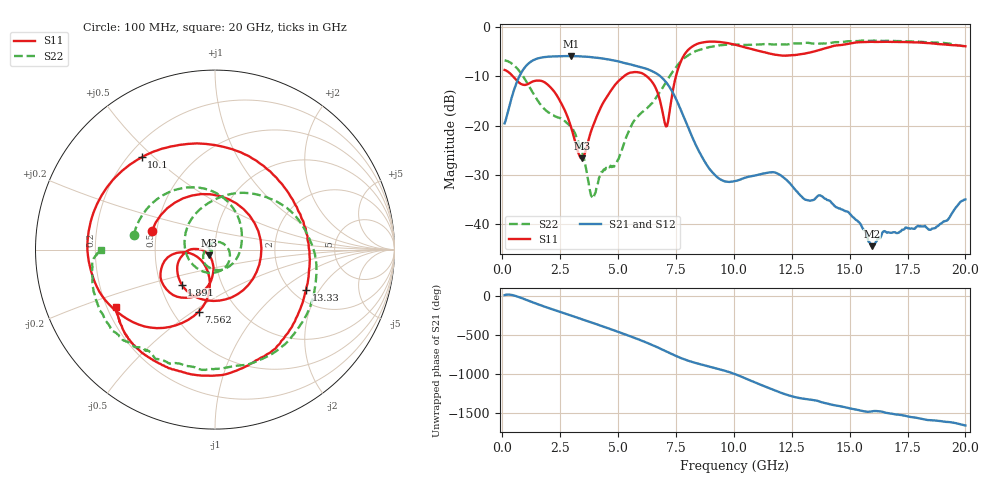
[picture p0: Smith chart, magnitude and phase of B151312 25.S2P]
!  2-Port S-parameters saved by WinCal
! VAR MeasName=S-Parameters (CALIBRATED_DATA) read from VNA (N5244A)
! VAR MeasDate=12/8/2015 5:45:19 PM
! VAR NAME=B151312 25
! VAR FILENAME=B151312 25.S2P
! VAR DATE=12/8/2015 5:45:19 PM
! VAR PHYS_PORTS=1,2
# Hz S DB R 50
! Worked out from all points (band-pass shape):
!   401 points, 100 MHz to 20 GHz, reference 50 ohm
!   highest |S21| = -5.89 dB at 2.986 GHz (marker M1); lowest = -44.4 dB at 15.97 GHz (marker M2)
!   |S21| within 3 dB of the highest: 869.3 MHz to 6.44 GHz (5.571 GHz wide, 152 % of centre)
!   lowest |S11| = -26.6 dB at 3.433 GHz (marker M3), VSWR 1.10, Z = 46.6 - j2.91 ohm
!   |S11| at or under -10 dB: 462.5 MHz to 5.25 GHz (4.788 GHz wide, 168 % of centre); 6.236 GHz to 7.499 GHz (1.263 GHz wide, 18.4 % of centre)
!   |S22| runs from -34.8 to -2.7 dB; largest |S21 - S12| = 0.0016
!   S11 on the Smith chart (normalised r, x): 100 MHz: 0.47, +0.11; 1.891 GHz: 0.64, -0.27; 7.562 GHz: 0.67, -0.53; 10.1 GHz: 0.25, +0.46; 13.33 GHz: 2.36, -1.53; 20 GHz: 0.24, -0.26
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1e8  -8.71 163.8  -19.54 10.3  -19.54 10.3  -6.75 169.8
4.98e8  -10.19 94.8  -12.88 5.5  -12.88 5.5  -7.73 129.1
9.4575e8  -11.75 1.6  -8.35 -40.4  -8.35 -40.4  -10.33 84.9
1.891e9  -11.41 -133.6  -6.06 -144.3  -6.06 -144.3  -16.96 1.3
2.3885e9  -14.12 -166.9  -5.93 165.8  -5.93 165.8  -18.34 -54.7
2.9855e9  -20.55 178.3  -5.89 106.9  -5.89 106.8  -20.36 -127.0
3.43325e9  -26.65 -138.0  -5.97 62.2  -5.96 62.2  -25.04 -172.2
3.881e9  -20.51 -95.3  -6.13 17.0  -6.13 17.0  -34.50 -160.4
4.82625e9  -12.00 -107.5  -6.79 -80.8  -6.78 -80.9  -28.31 117.1
5.72175e9  -9.12 -141.0  -7.82 -178.0  -7.81 -178.0  -18.81 -61.1
6.7665e9  -14.15 -175.4  -9.76 53.7  -9.77 53.7  -13.43 129.1
7.11475e9  -20.08 -130.4  -11.45 5.3  -11.43 5.3  -10.86 87.1
7.5625e9  -8.92 -104.8  -15.21 -55.9  -15.18 -55.7  -7.79 46.0
8.7565e9  -3.06 -172.5  -27.39 -169.8  -27.40 -170.1  -4.28 -27.4
1.005e10  -3.59 130.8  -31.26 80.0  -31.28 79.5  -3.54 -70.7
1.009975e10  -3.65 128.5  -31.19 74.4  -31.23 73.9  -3.54 -71.9
1.13435e10  -5.13 70.2  -29.66 -77.9  -29.72 -77.8  -3.44 -95.4
1.33335e10  -5.12 -23.9  -35.19 112.8  -35.20 113.3  -3.31 -120.5
1.338325e10  -5.07 -26.0  -35.13 110.5  -35.09 111.1  -3.34 -121.0
1.597025e10  -3.00 -100.7  -44.44 -35.3  -44.48 -35.5  -2.79 -146.1
1.67165e10  -3.02 -113.7  -41.67 -61.1  -41.53 -60.8  -2.78 -152.5
2e10  -3.91 -149.8  -34.96 144.0  -34.98 142.9  -3.92 -179.8
